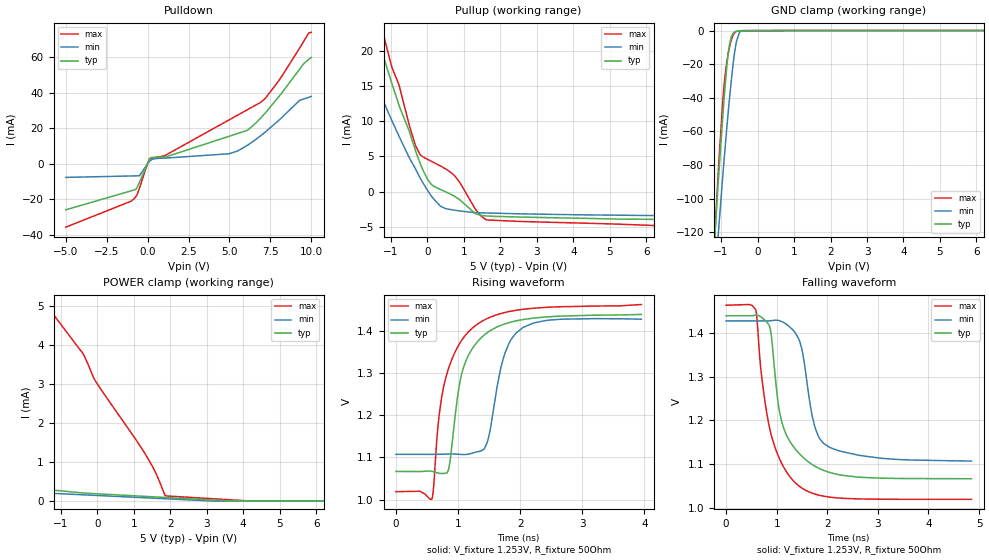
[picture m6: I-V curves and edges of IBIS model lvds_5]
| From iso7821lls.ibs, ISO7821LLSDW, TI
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|   lvds_5 Model
[Model]   lvds_5
Model_type   3-state
Polarity   Non-Inverting
Vmeas = 1.253
Vref = 1.253
Cref = 2pF
Rref = 50
|   typ   min   max
|   (nom PVT)   (fast PVT)   (slow PVT)
C_comp   4.937e-12   4.148e-12   5.615e-12
| Where nom  PVT is Nominal Process, 5V, 27C
|   Fast PVT is Strong Process,  5.5V, -55C
|   Slow PVT is Weak Process,   4.5V, 150C
[Voltage Range]   5   4.5   5.5
|Junction Temperature
[Temperature Range]   27   150   -55
[Pullup Reference]   5   4.5   5.5
[Pulldown Reference]   0   0   0
[Power Clamp Reference]   5   4.5   5.5
[GND Clamp Reference]   0   0   0
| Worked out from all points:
|   slope of the pulldown table from 0 to 0.75 V, typ, clamps not added: 211 ohm
|   slope of the pullup table from 0 to 0.75 V, typ, clamps not added: 303 ohm
|   GND clamp passes 1 mA (typ) near -0.64 V on its own axis
|   falling waveform, V_fixture 1.253V, R_fixture 50Ohm: 20-80 % time 404ps typ, 302ps min, 426ps max; typ from 1.44 V to 1.07 V
|   rising waveform, V_fixture 1.253V, R_fixture 50Ohm: 20-80 % time 349ps typ, 276ps min, 399ps max; typ from 1.07 V to 1.44 V
[Pulldown]
|   Voltage   I(typ)   I(min)   I(max)
-5V       -25.95mA   -7.687mA   -35.73mA
-1.008V   -15.26mA   -6.882mA   -21.11mA
-635mV    -13.2mA    -6.806mA   -17.21mA
-500mV    -10.48mA   -6.779mA   -13.82mA
110mV     2.115mA    1.231mA    2.913mA
1.02V     3.714mA    3.176mA    4.425mA
4.972V    15.46mA    5.636mA    24.69mA
6.085V    18.81mA    10.31mA    30.4mA
7.181V    28.5mA     17.79mA    36.73mA
9.287V    53.25mA    35.73mA    65.14mA
9.85V     58.81mA    37.48mA    73.69mA
10V       59.94mA    37.94mA    74.08mA
[GND Clamp]
|   Voltage   I(typ)   I(min)   I(max)
-5V       -1.683A    -1.481A    -1.922A
-1.288V   -162.9mA   -183.7mA   -169.4mA
-1.095V   -96.08mA   -126.3mA   -90.93mA
-1.062V   -85.19mA   -116.8mA   -78.58mA
-919mV    -41.23mA   -77.42mA   -32.82mA
-850mV    -23.23mA   -59.69mA   -19.72mA
-785mV    -10.39mA   -44.01mA   -11.53mA
-720.5mV  -3.773mA   -29.76mA   -5.645mA
-581mV    -401.1uA   -6.591mA   -553.1uA
-495.5mV  -136.3uA   -1.186mA   -151.7uA
-347mV    -80.83uA   -96.29uA   -89.83uA
10V       0A         0A         0A
[Pullup]
|   Voltage   I(typ)   I(min)   I(max)
-5V       75.4mA     58.14mA    85.82mA
-3.045V   50.04mA    35.28mA    59.26mA
-1.99V    32.44mA    22.14mA    38.26mA
-1.034V   16.33mA    10.77mA    18.81mA
-770.5mV  12.12mA    7.77mA     14.98mA
-336mV    5.941mA    3.31mA     6.672mA
-204mV    4.064mA    1.977mA    5.292mA
100mV     1.059mA    -566.2uA   4.323mA
505.5mV   -49.02uA   -2.42mA    3.2mA
740mV     -657.8uA   -2.634mA   2.276mA
1.617V    -3.461mA   -3.036mA   -4.024mA
10V       -4.102mA   -3.6mA     -5.508mA
[POWER Clamp]
|   Voltage   I(typ)   I(min)   I(max)
-5V       13.36mA    2.167mA    35.57mA
-4.868V   8.38mA     808uA      29.03mA
-4.758V   5.049mA    467.3uA    23.76mA
-4.695V   3.721mA    402uA      20.88mA
-4.649V   3.079mA    378uA      18.87mA
-4.59V    2.602mA    361.4uA    16.46mA
-4.475V   2.253mA    347.3uA    12.77mA
-2.646V   711.8uA    263uA      6.992mA
-1.75V    342.6uA    222.9uA    5.477mA
-402mV    210.9uA    162.6uA    3.795mA
1.871V    93.49uA    60.75uA    140.8uA
10V       0A         0A         0A
[Ramp]
R_load = 50
|   typ   min   max
dV/dt_r   0.114751/7.00717e-10  0.0985309/9.08708e-10   0.137925/5.73941e-10
dV/dt_f   0.223149/4.03833e-10   0.191897/2.9906e-10   0.265747/4.25926e-10
[Falling Waveform]
V_fixture = 1.253V
V_fixture_min = 1.267V
V_fixture_max = 1.241V
R_fixture = 50Ohm
|   Time   V(typ)   V(min)   V(max)
0s        1.439V     1.427V     1.463V
585ps     1.44V      1.427V     1.453V
709.3ps   1.435V     1.427V     1.294V
846.7ps   1.418V     1.427V     1.19V
1.015ns   1.252V     1.428V     1.124V
1.099ns   1.197V     1.426V     1.102V
1.459ns   1.123V     1.379V     1.049V
1.701ns   1.099V     1.211V     1.034V
1.93ns    1.086V     1.147V     1.027V
4.85ns    1.067V     1.107V     1.02V
[Rising Waveform]
V_fixture = 1.253V
V_fixture_min = 1.267V
V_fixture_max = 1.241V
R_fixture = 50Ohm
|   Time   V(typ)   V(min)   V(max)
0s        1.066V     1.107V     1.019V
579.3ps   1.067V     1.107V     1.001V
695.2ps   1.062V     1.107V     1.199V
829.3ps   1.065V     1.108V     1.302V
1.034ns   1.281V     1.107V     1.371V
1.266ns   1.365V     1.111V     1.41V
1.472ns   1.395V     1.137V     1.429V
1.724ns   1.414V     1.332V     1.442V
2.038ns   1.426V     1.406V     1.45V
3.95ns    1.438V     1.427V     1.462V
